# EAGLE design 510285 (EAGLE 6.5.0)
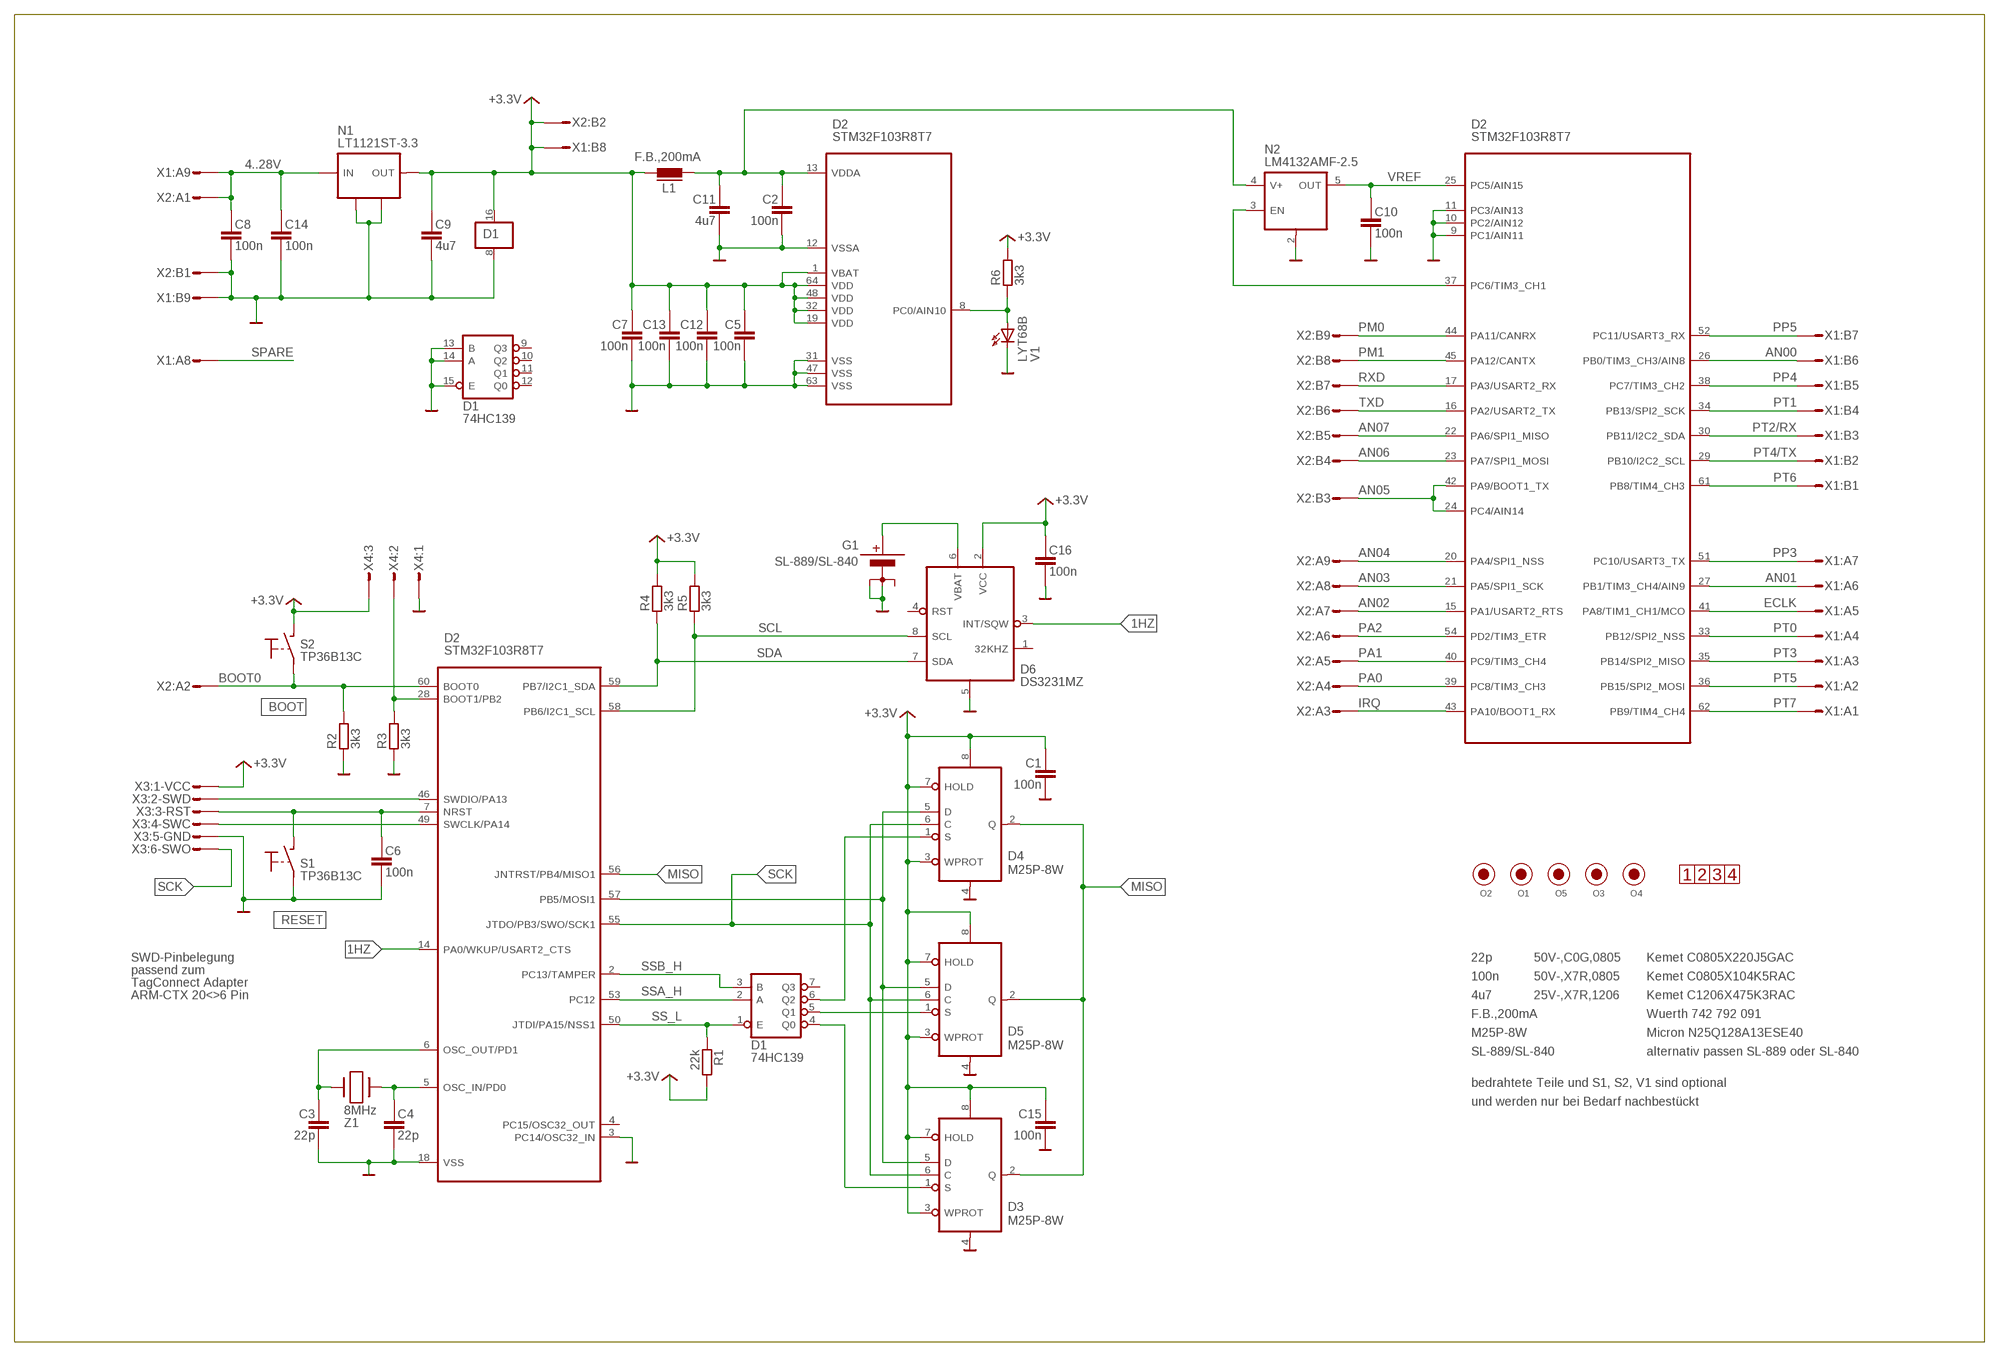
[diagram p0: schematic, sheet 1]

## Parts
C1  100n  C-EU-H-0805  [C0805]
C2  100n  C-EU-H-0805  [C0805]
C3  22p  C-EU-H-0805  [C0805]
C4  22p  C-EU-H-0805  [C0805]
C5  100n  C-EU-H-0805  [C0805]
C6  100n  C-EU-H-0805  [C0805]
C7  100n  C-EU-H-0805  [C0805]
C8  100n  C-EU-H-0805  [C0805]
C9  4u7  C-EU-H-1206  [C1206]
C10  100n  C-EU-H-0805  [C0805]
C11  4u7  C-EU-H-1206  [C1206]
C12  100n  C-EU-H-0805  [C0805]
C13  100n  C-EU-H-0805  [C0805]
C14  100n  C-EU-H-0805  [C0805]
C15  100n  C-EU-H-0805  [C0805]
C16  100n  C-EU-H-0805  [C0805]
D1  74HC139  74HC139D  [SO-16]
D2  STM32F103R8T7  [LQFP-10X10-64]
D3  M25P-8W  M25-8W  [SO-8-208MIL]
D4  M25P-8W  M25-8W  [SO-8-208MIL]
D5  M25P-8W  M25-8W  [SO-8-208MIL]
D6  DS3231MZ  [SO-8]
G1  SL-889/SL-840  BATTERIE-3MINUS  [SL-889/840-510285]
L1  F.B.,200mA  EMV-FERRIT-0805  [L0805]
N1  LT1121ST-3.3  [SOT-223]
N2  LM4132AMF-2.5  [MF05A]
O1  FIDUCIAL  [FIDUCIAL-1]
O2  FIDUCIAL  [FIDUCIAL-1]
O3  FIDUCIAL  [FIDUCIAL-1]
O4  FIDUCIAL  [FIDUCIAL-1]
O5  FIDUCIAL  [FIDUCIAL-1]
O6  1234-15  [1234-15]
R1  22k  R_0805  [R0805]
R2  3k3  R_0805  [R0805]
R3  3k3  R_0805  [R0805]
R4  3k3  R_0805  [R0805]
R5  3k3  R_0805  [R0805]
R6  3k3  R_0805  [R0805]
S1  TP36B13C  [TP36]
S2  TP36B13C  [TP36]
V1  LYT68B  LYT679-CO  [PLCC-2]
X1  1022-A-xx1-018  MODU-2X09-MVSS  [1022-A-XX1-018]
X2  1022-A-xx1-018  MODU-2X09-MVSS  [1022-A-XX1-018]
X3  SLR2-2x03  TAG-CONNECT-6M-SLR  [TAG-CONNECT-6-SLR]
X4  MODU-1X03-MV  [MODU-1X03-XV]
Z1  8MHz  HC-49/US-0.7  [HC-49/US-0.7]

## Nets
1HZ: D2.14(PA0/WKUP/USART2_CTS:I/O) D6.3(INT/SQW)
4..28V: C8.1 C14.1 N1.1(IN) X1.A9 X2.A1
+3.3V: C1.1 C5.1 C7.1 C9.1 C12.1 C13.1 C15.1 C16.1 D1.16(VDD) D2.1(VBAT:PWR) D2.19(VDD@19:VDD) D2.32(VDD@32:VDD) D2.48(VDD@48:VDD) D2.64(VDD@64:VDD) D3.3(WPROT) D3.7(HOLD) D3.8(VDD) D4.3(WPROT) D4.7(HOLD) D4.8(VDD) D5.3(WPROT) D5.7(HOLD) D5.8(VDD) D6.2(VCC) L1.1 N1.3(OUT) R1.2 R4.2 R5.2 R6.2 S2.1(NO1) X1.B8 X2.B2 X3.1 X4.3
AN00: D2.26(PB0/TIM3_CH3/AIN8:I/O) X1.B6
AN01: D2.27(PB1/TIM3_CH4/AIN9:I/O) X1.A6
AN02: D2.15(PA1/USART2_RTS:I/O) X2.A7
AN03: D2.21(PA5/SPI1_SCK:I/O) X2.A8
AN04: D2.20(PA4/SPI1_NSS:I/O) X2.A9
AN05: D2.24(PC4/AIN14:I/O) D2.42(PA9/BOOT1_TX:I/O) X2.B3
AN06: D2.23(PA7/SPI1_MOSI:I/O) X2.B4
AN07: D2.22(PA6/SPI1_MISO:I/O) X2.B5
BOOT0: D2.60(BOOT0:IN) R2.2 S2.2(NO2) X2.A2
BOOT1: D2.28(BOOT1/PB2:I/O) R3.2 X4.2
ECLK: D2.41(PA8/TIM1_CH1/MCO:I/O) X1.A5
GND: C1.2 C2.2 C3.2 C4.2 C5.2 C6.2 C7.2 C8.2 C9.2 C10.2 C11.2 C12.2 C13.2 C14.2 C15.2 C16.2 D1.8(GND) D1.13(B) D1.14(A) D1.15(E) D2.3(PC14/OSC32_IN:IN) D2.9(PC1/AIN11:I/O) D2.10(PC2/AIN12:I/O) D2.11(PC3/AIN13:I/O) D2.12(VSSA:PWR) D2.18(VSS@18:VSS) D2.31(VSS@31:VSS) D2.47(VSS@47:VSS) D2.63(VSS@63:VSS) D3.4(GND) D4.4(GND) D5.4(GND) D6.5(GND) G1.-2 G1.-BELP(-3) N1.2(GND) N1.4(GND) N2.2(GND) R2.1 R3.1 S1.2(NO2) V1.C X1.B9 X2.B1 X3.5 X4.1
IRQ: D2.43(PA10/BOOT1_RX:I/O) X2.A3
LED: D2.8(PC0/AIN10:I/O) R6.1 V1.A
MISO: D2.56(JNTRST/PB4/MISO1:I/O) D3.2(Q) D4.2(Q) D5.2(Q)
MOSI: D2.57(PB5/MOSI1:I/O) D3.5(D) D4.5(D) D5.5(D)
OSCIN: C4.1 D2.5(OSC_IN/PD0:IN) Z1.2
OSCOUT: C3.1 D2.6(OSC_OUT/PD1:OUT) Z1.1
PA0: D2.39(PC8/TIM3_CH3:I/O) X2.A4
PA1: D2.40(PC9/TIM3_CH4:I/O) X2.A5
PA2: D2.54(PD2/TIM3_ETR:I/O) X2.A6
PM0: D2.44(PA11/CANRX:I/O) X2.B9
PM1: D2.45(PA12/CANTX:I/O) X2.B8
PP3: D2.51(PC10/USART3_TX:I/O) X1.A7
PP4: D2.38(PC7/TIM3_CH2:I/O) X1.B5
PP5: D2.52(PC11/USART3_RX:I/O) X1.B7
PT0: D2.33(PB12/SPI2_NSS:I/O) X1.A4
PT1: D2.34(PB13/SPI2_SCK:I/O) X1.B4
PT2/RX: D2.30(PB11/I2C2_SDA:I/O) X1.B3
PT3: D2.35(PB14/SPI2_MISO:I/O) X1.A3
PT4/TX: D2.29(PB10/I2C2_SCL:I/O) X1.B2
PT5: D2.36(PB15/SPI2_MOSI:I/O) X1.A2
PT6: D2.61(PB8/TIM4_CH3:I/O) X1.B1
PT7: D2.62(PB9/TIM4_CH4:I/O) X1.A1
RESET_L: C6.1 D2.7(NRST:I/O) S1.1(NO1) X3.3
RXD: D2.17(PA3/USART2_RX:I/O) X2.B7
SCK: D2.55(JTDO/PB3/SWO/SCK1:I/O) D3.6(C) D4.6(C) D5.6(C) X3.6
SCL: D2.58(PB6/I2C1_SCL:I/O) D6.8(SCL) R5.1
SDA: D2.59(PB7/I2C1_SDA:I/O) D6.7(SDA) R4.1
SPARE: X1.A8
SS0_L: D1.4(Q0) D3.1(S)
SS1_L: D1.5(Q1) D5.1(S)
SS2_L: D1.6(Q2) D4.1(S)
SS_L: D1.1(E) D2.50(JTDI/PA15/NSS1:I/O) R1.1
SSA_H: D1.2(A) D2.53(PC12:I/O)
SSB_H: D1.3(B) D2.2(PC13/TAMPER:I/O)
SWCLK: D2.49(SWCLK/PA14:I/O) X3.4
SWDIO: D2.46(SWDIO/PA13:I/O) X3.2
TXD: D2.16(PA2/USART2_TX:I/O) X2.B6
VBAT [VBAT]: D6.6(VBAT) G1.+
VDDA: C2.1 C11.1 D2.13(VDDA:I/O) L1.2 N2.4(V+)
VREF: C10.1 D2.25(PC5/AIN15:I/O) N2.5(OUT)
VREFEN_H: D2.37(PC6/TIM3_CH1:I/O) N2.3(EN)
Unconnected: D1.7(Q3) D1.9(Q3) D1.10(Q2) D1.11(Q1) D1.12(Q0) D2.4(PC15/OSC32_OUT:OUT) D6.1(32KHZ) D6.4(RST) G1.-1 O1.F O2.F O3.F O4.F O5.F

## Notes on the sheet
- BOOT
- RESET
- SWD-Pinbelegung | 22p | 50V-,C0G,0805 | Kemet C0805X220J5GAC
- passend zum
- 100n | 50V-,X7R,0805 | Kemet C0805X104K5RAC
- TagConnect Adapter
- ARM-CTX 20<>6 Pin | 4u7 | 25V-,X7R,1206 | Kemet C1206X475K3RAC
- F.B.,200mA | Wuerth 742 792 091
- M25P-8W | Micron N25Q128A13ESE40
- SL-889/SL-840 | alternativ passen SL-889 oder SL-840
- bedrahtete Teile und S1, S2, V1 sind optional
- und werden nur bei Bedarf nachbestückt

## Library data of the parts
C1-C16 = din-C:C-EU-H-
D1 = din-D:74*139
D2 = din-D:STM32F103R
D3-D5 = din-D:M25*
D6 = din-D:DS3231*Z
G1 = din-G:BATTERIE-3MINUS
L1 = din-L:EMV-FERRIT: 0805: WE742792091, 1500Ohm@100MHz, 0.55Ohm, 0.2A
N1 = din-N:LT1121*
N2 = din-N:LM4132
O1-O5 = din-O:FIDUCIAL
O6 = din-O:1234
R1-R6 = din-R:R_
S1 S2 = din-S:TP36
V1 = din-V:L*T679-CO
X1 X2 = din-X:MODU-2X09-M
X3 = din-X:TAG-CONNECT-6M
X4 = din-X:MODU-1X03-M
Z1 = din-Z:HC-49/US

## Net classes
1 VBAT: clearance 0.53 mm to class 0

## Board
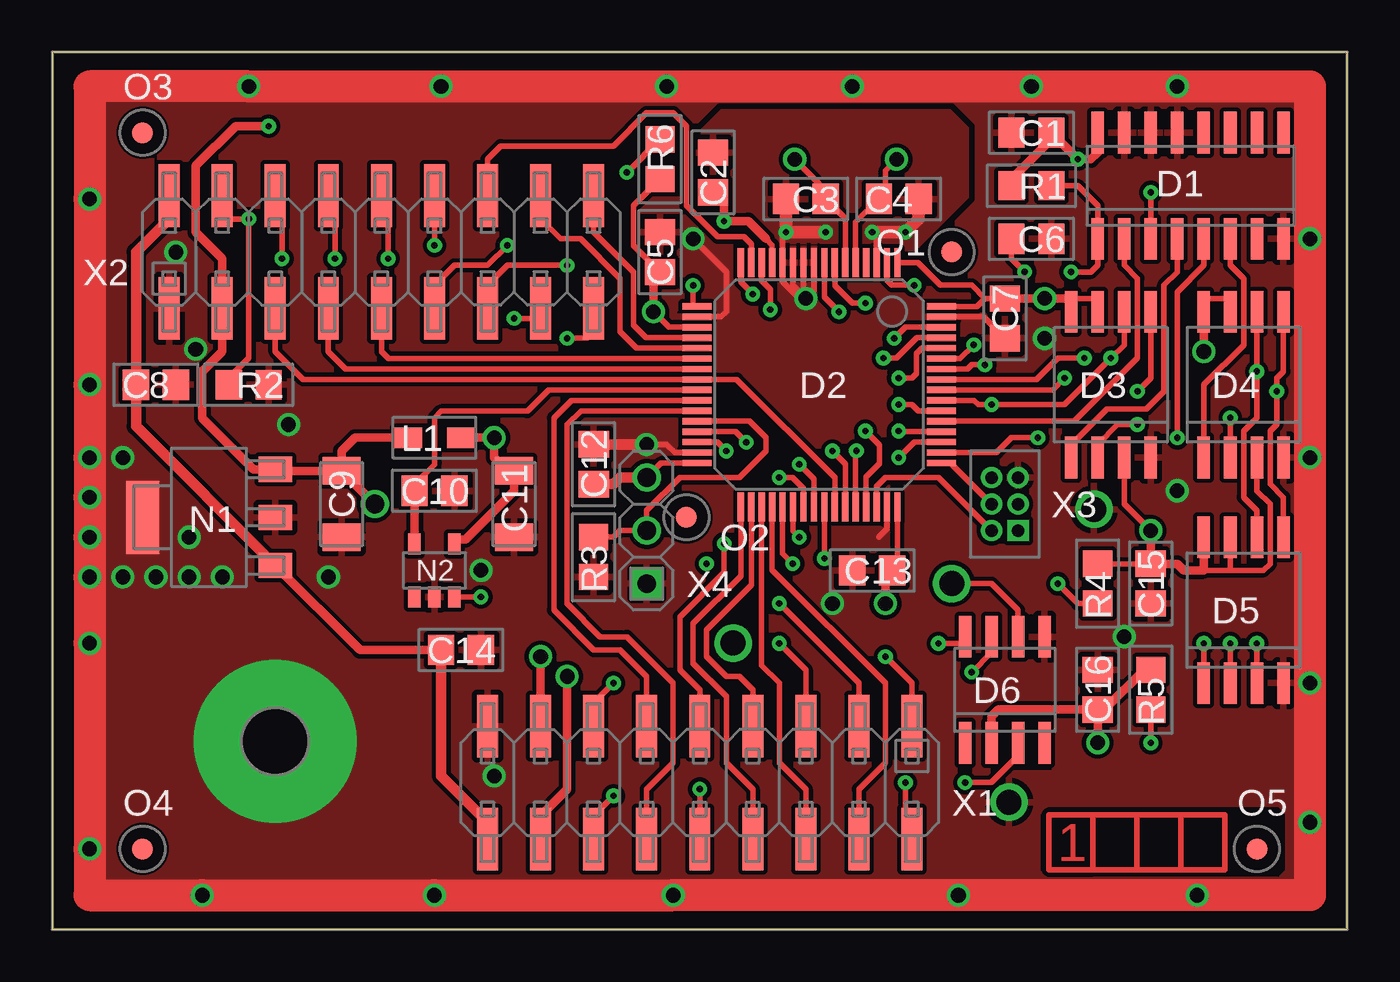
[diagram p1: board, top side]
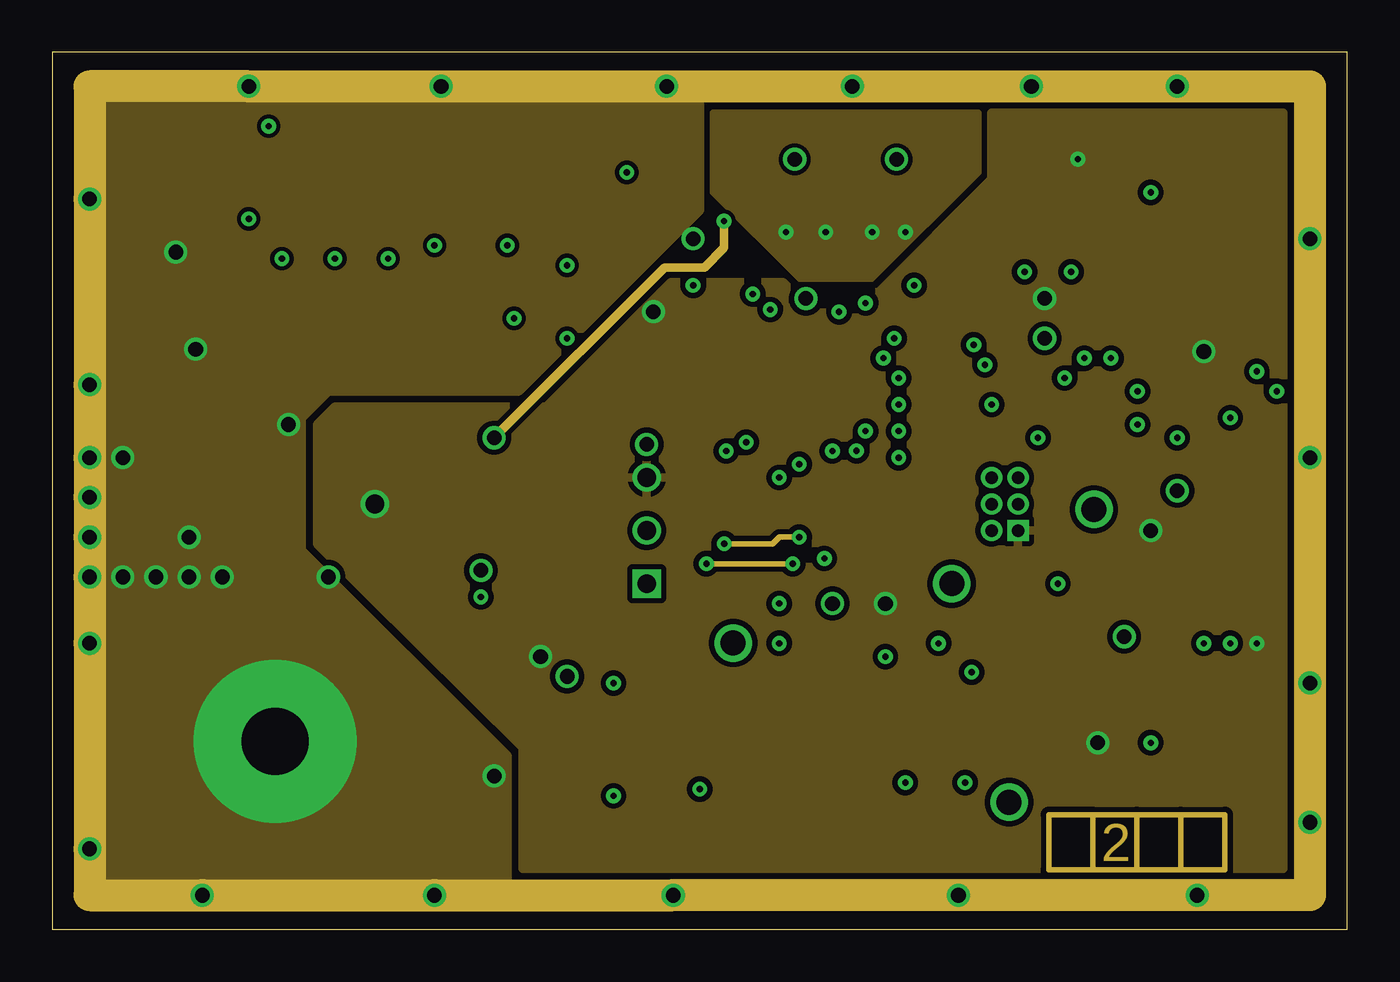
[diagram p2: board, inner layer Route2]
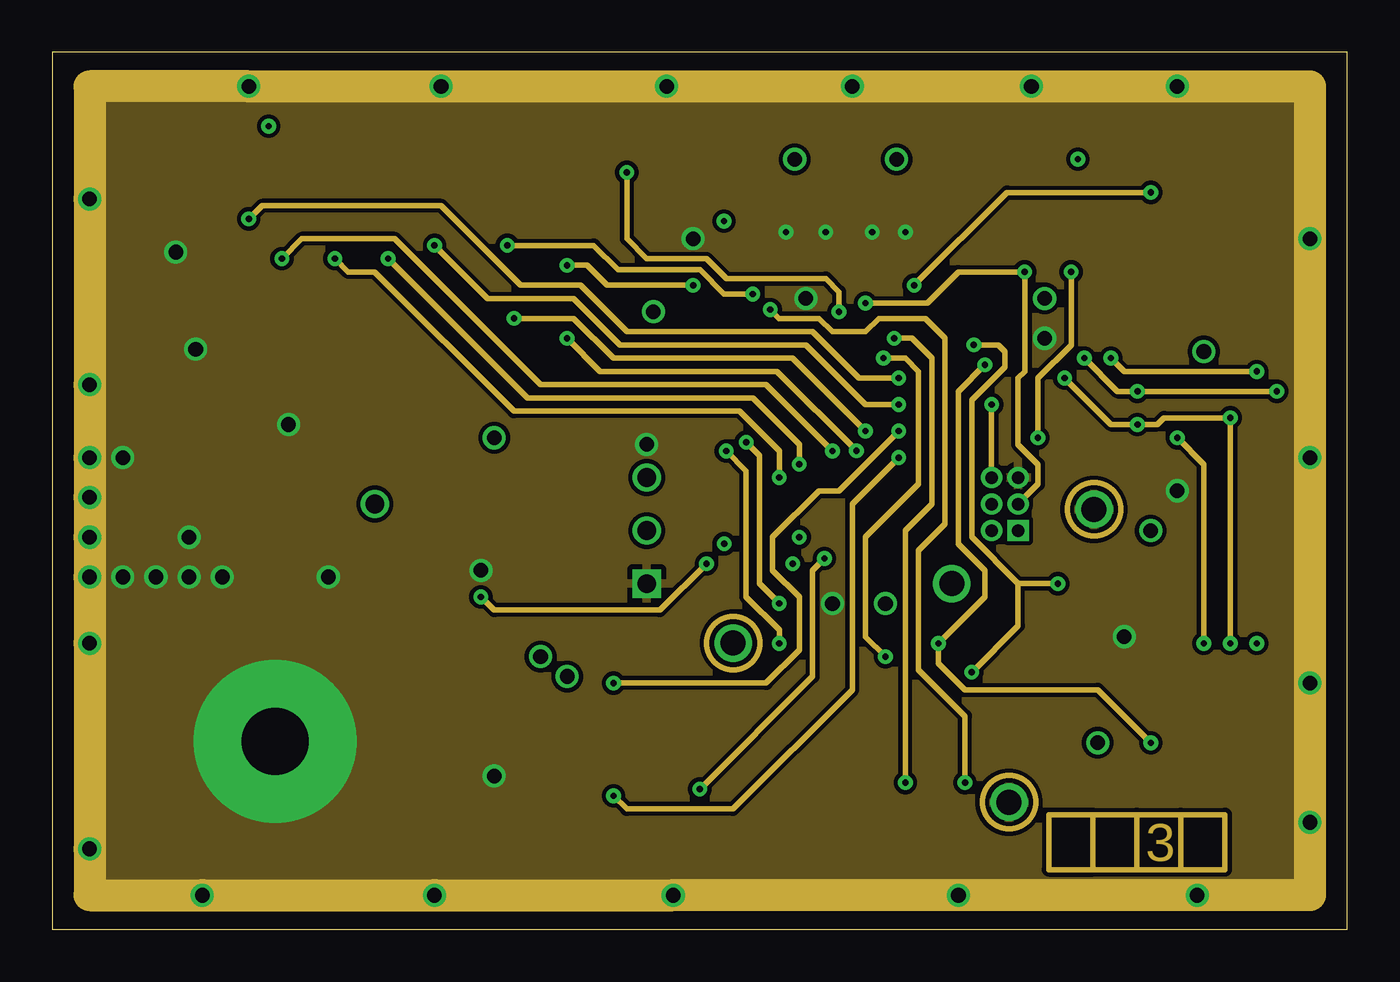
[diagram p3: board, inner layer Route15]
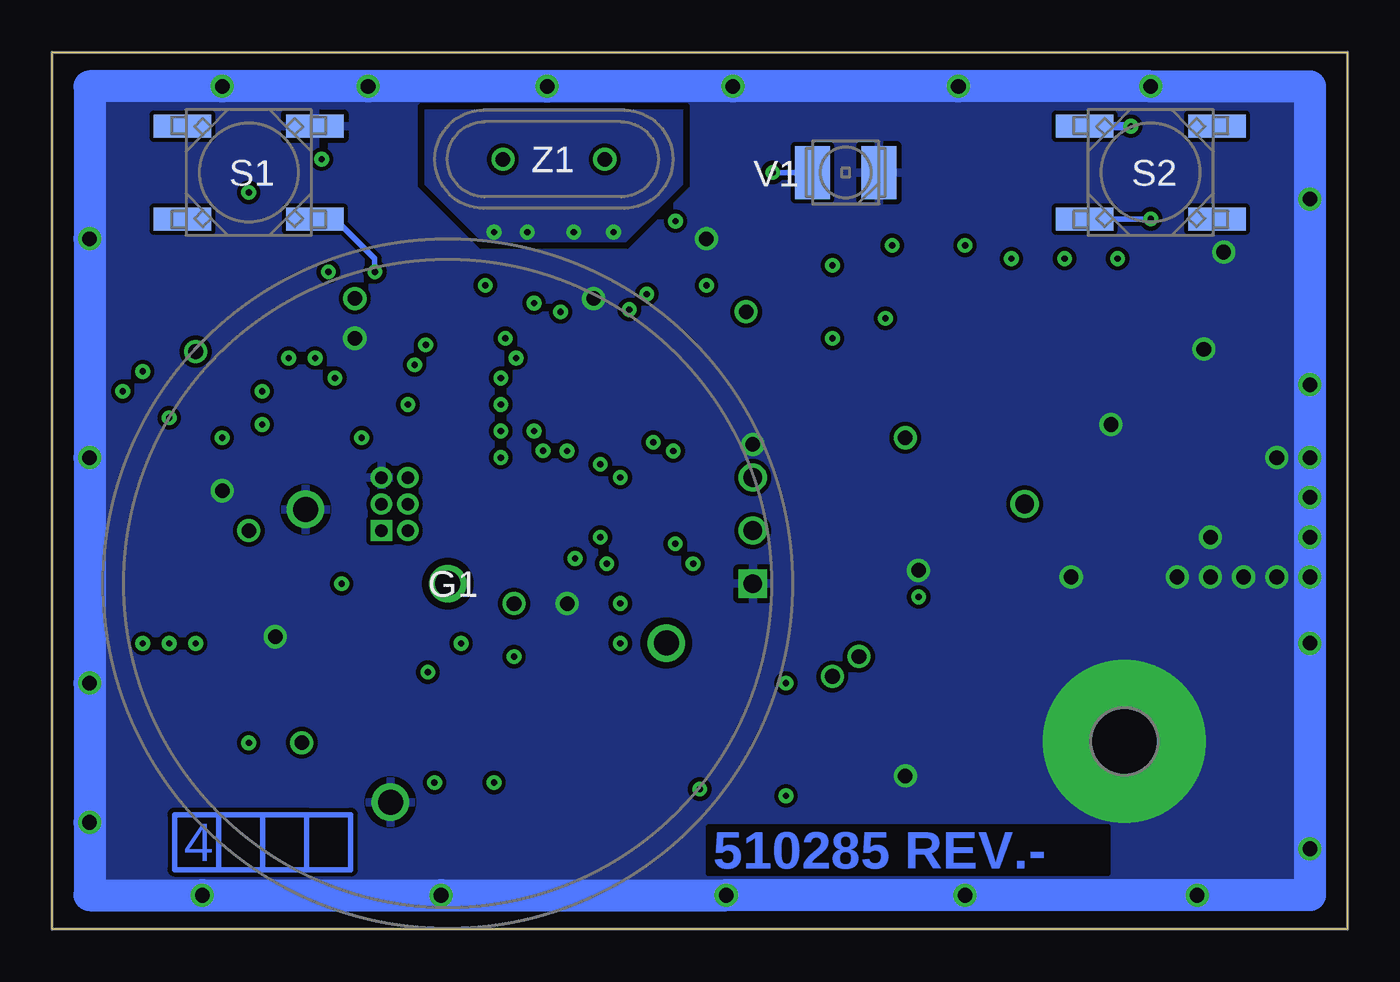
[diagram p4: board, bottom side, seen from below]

Size 62 x 42 mm. Coordinates in mm from the lower left corner, seen from the top.
Outline: 0,0 62,0 62,42 0,42 0,0
Copper layers (1+2*15+16): Top 0.018mm / dielectric 0.156mm / Route2 0.035mm / dielectric 1.2mm / Route15 0.035mm / dielectric 0.156mm / Bottom 0.018mm
Design rules "default *": minimum track width 10mil, minimum drill 0.3mm, track to track 8mil, track to pad 8mil, pad to pad 0.192mm, via to via 8mil, smd to smd 0.192mm, copper to edge 0.6mm, drill to drill 8mil, minimum pad ring 8mil, minimum via ring 8mil, stop-mask expansion 4mil, vias tented up to drill 0mil, thermal gap 10mil
tKeepout: area 2,4 to 14,10; area 5,3.2 to 16.4,14.6; area 50.1,3.9 to 60.2,8.9
tRestrict: 23 lines
bRestrict: 10 lines

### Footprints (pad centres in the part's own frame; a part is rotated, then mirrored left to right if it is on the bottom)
C0805 = smd 1.255 x 1.45: 1 -0.953,0; 2 0.953,0
C1206 = smd 1.325 x 1.8: 1 -1.587,0; 2 1.587,0
SO-16 = smd 0.6 x 2: 1 -4.445,-2.54; 2 -3.175,-2.54; 3 -1.905,-2.54; 4 -0.635,-2.54; 5 0.635,-2.54; 6 1.905,-2.54; 7 3.175,-2.54; 8 4.445,-2.54; 9 4.445,2.54; 10 3.175,2.54; 11 1.905,2.54; 12 0.635,2.54; 13 -0.635,2.54; 14 -1.905,2.54; 15 -3.175,2.54; 16 -4.445,2.54
LQFP-10X10-64 = smd 1.4 x 0.3: 1 -5.85,3.75; 2 -5.85,3.25; 3 -5.85,2.75; 4 -5.85,2.25; 5 -5.85,1.75; 6 -5.85,1.25; 7 -5.85,0.75; 8 -5.85,0.25; 9 -5.85,-0.25; 10 -5.85,-0.75; 11 -5.85,-1.25; 12 -5.85,-1.75; 13 -5.85,-2.25; 14 -5.85,-2.75; 15 -5.85,-3.25; 16 -5.85,-3.75; 33 5.85,-3.75; 34 5.85,-3.25; 35 5.85,-2.75; 36 5.85,-2.25; 37 5.85,-1.75; 38 5.85,-1.25; 39 5.85,-0.75; 40 5.85,-0.25; 41 5.85,0.25; 42 5.85,0.75; 43 5.85,1.25; 44 5.85,1.75; 45 5.85,2.25; 46 5.85,2.75; 47 5.85,3.25; 48 5.85,3.75 | smd 0.3 x 1.4: 17 -3.75,-5.85; 18 -3.25,-5.85; 19 -2.75,-5.85; 20 -2.25,-5.85; 21 -1.75,-5.85; 22 -1.25,-5.85; 23 -0.75,-5.85; 24 -0.25,-5.85; 25 0.25,-5.85; 26 0.75,-5.85; 27 1.25,-5.85; 28 1.75,-5.85; 29 2.25,-5.85; 30 2.75,-5.85; 31 3.25,-5.85; 32 3.75,-5.85; 49 3.75,5.85; 50 3.25,5.85; 51 2.75,5.85; 52 2.25,5.85; 53 1.75,5.85; 54 1.25,5.85; 55 0.75,5.85; 56 0.25,5.85; 57 -0.25,5.85; 58 -0.75,5.85; 59 -1.25,5.85; 60 -1.75,5.85; 61 -2.25,5.85; 62 -2.75,5.85; 63 -3.25,5.85; 64 -3.75,5.85
SO-8-208MIL = smd 0.6 x 2: 1 -1.905,-3.493; 2 -0.635,-3.493; 3 0.635,-3.493; 4 1.905,-3.493; 5 1.905,3.493; 6 0.635,3.493; 7 -0.635,3.493; 8 -1.905,3.493
SO-8 = smd 0.6 x 2: 1 -1.905,-2.54; 2 -0.635,-2.54; 3 0.635,-2.54; 4 1.905,-2.54; 5 1.905,2.54; 6 0.635,2.54; 7 -0.635,2.54; 8 -1.905,2.54
SL-889/840-510285 = drill 1.2: + 0,0; -1 10.465,-2.845; -2 -2.743,-10.465; -BELP -6.807,3.556
L0805 = smd 1.34 x 1: 1 -1.27,0; 2 1.27,0
SOT-223 = smd 1.2 x 1.6: 1 -2.3,-3.175; 2 0,-3.175; 3 2.3,-3.175 | smd 3.5 x 1.6: 4 0,3.175
MF05A = smd 0.6 x 1: 1 -0.953,-1.27; 2 0,-1.27; 3 0.953,-1.27; 4 0.953,1.27; 5 -0.953,1.27
FIDUCIAL-1 = smd 1 x 1: F 0,0
R0805 = smd 1.255 x 1.4: 1 -0.953,0; 2 0.953,0
TP36 = smd 1.1 x 2.75: 1 -2.223,-3.175; 2 2.223,-3.175; 3 2.223,3.175; 4 -2.223,3.175
PLCC-2 = smd 2.54 x 1.675: A 0,1.587; C 0,-1.587
1022-A-XX1-018 = smd 1 x 3: A1 -10.16,2.7; A2 -7.62,2.7; A3 -5.08,2.7; A4 -2.54,2.7; A5 0,2.7; A6 2.54,2.7; A7 5.08,2.7; A8 7.62,2.7; A9 10.16,2.7; B1 -10.16,-2.7; B2 -7.62,-2.7; B3 -5.08,-2.7; B4 -2.54,-2.7; B5 0,-2.7; B6 2.54,-2.7; B7 5.08,-2.7; B8 7.62,-2.7; B9 10.16,-2.7
TAG-CONNECT-6-SLR = drill 0.6 pad 1.016 square: 1 -1.27,-0.635 | drill 0.6 pad 1.016: 2 -1.27,0.635; 3 0,-0.635; 4 0,0.635; 5 1.27,-0.635; 6 1.27,0.635
MODU-1X03-XV = drill 0.9 square: 1 -2.54,0 | drill 0.9: 2 0,0; 3 2.54,0
HC-49/US-0.7 = drill 0.7 pad 1.1: 1 -2.44,0; 2 2.44,0

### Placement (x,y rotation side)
C1  46.88,38.14 180 top
C2  31.64,36.24 90 top
C3  36.08,34.97 180 top
C4  40.52,34.97 0 top
C5  29.09,32.43 90 top
C6  46.88,33.06 0 top
C7  45.61,29.26 270 top
C8  4.96,26.08 0 top
C9  13.86,20.36 270 top
C10  18.3,21 0 top
C11  22.11,20.36 270 top
C12  25.92,22.27 90 top
C13  39.26,17.19 180 top
C14  19.57,13.38 0 top
C15  52.59,16.55 270 top
C16  50.05,11.47 90 top
D1  54.5,35.61 0 top
D2  36.72,26.08 270 top
D3  50.69,26.08 0 top
D4  57.03,26.08 0 top
D5  57.03,15.29 0 top
D6  45.61,11.47 0 top
G1  43.06,16.55 0 bottom
L1  18.3,23.54 0 top
N1  7.5,19.73 90 top
N2  18.3,17.19 0 top
O1  43.06,32.43 0 top
O2  30.36,19.73 0 top
O3  4.33,38.14 0 top
O4  4.33,3.86 0 top
O5  57.67,3.86 0 top
O6  51.92,4.17 0 top
R1  46.88,35.61 180 top
R2  9.41,26.08 180 top
R3  25.92,17.82 90 top
R4  50.05,16.55 90 top
R5  52.59,11.47 90 top
R6  29.09,36.88 270 top
S1  52.59,36.24 90 bottom
S2  9.41,36.24 270 bottom
V1  24.02,36.24 90 bottom
X1  31,7.03 180 top
X2  15.76,32.43 0 top
X3  45.61,20.36 90 top
X4  28.46,19.09 90 top
Z1  37.98,36.88 180 bottom

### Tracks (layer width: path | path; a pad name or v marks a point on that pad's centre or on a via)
1HZ  (via drill 0.3)
  Top 0.254: D6.3 46.24,8.3 44.97,7.03 v43.7,7.03 | D2.14 33.97,31.05 34.38,30.64 v34.38,29.67
  Route15 0.254: v43.7,7.03 43.7,10.21 41.48,12.43 41.48,18.14 42.75,19.41 42.75,28.3 41.8,29.26 39.57,29.26 38.94,28.62 37.35,28.62 36.72,29.26 34.8,29.26 v34.38,29.67
4..28V
  Top 0.406: N1.1 14.73,13.38 C14.1
  Top 0.508: X2.A1 5.6,34.02 4.01,32.43 C8.1 4.01,24.1 N1.1 | X1.A9 20.84,5.12 18.62,7.35 C14.1
+3.3V  (via drill 0.3, 0.7, 0.9)
  Top 0.254: D2.48 40.47,17.45 C13.1 | D3.3 51.32,20.36 v52.59,19.09 | D2.64 44.27,29.83 44.65,30.21 | 44.65,30.21 C7.1 | D3.7 50.05,30.21 48.78,30.21 | D2.1 41.44,31.93 42.53,30.84 44.02,30.84 44.65,30.21 | D4.3 57.67,21 58.3,20.36 58.3,17.51 57.99,17.19 56.4,17.19 | 56.4,17.19 D5.7 | D4.7 56.4,30.21 55.13,30.21 D4.8 | 55.13,17.19 56.4,17.19 | D5.3 v57.67,13.7 | R4.2 C15.1 | D2.32 29.16,22.33 X4.3 | D2.19 29.52,28.83 v28.78,29.57 | R6.2 27.82,34.65 27.82,32.75 C5.1
  Top 0.406: v52.59,19.09 C15.1 53.86,17.51 54.18,17.19 55.13,17.19 D5.8 | v39.89,15.6 39.89,16.87 C13.1 | D6.2 44.97,10.21 45.29,10.52 C16.1 | C7.1 v47.51,30.21 48.78,30.21 D3.8 | R1.2 45.92,35.92 47.83,37.83 C1.1 v49.1,36.88 49.73,36.88 50.05,37.19 D1.16 | v55.13,27.67 D4.8 | C16.1 v50.05,8.94 | v28.78,29.57 28.78,31.16 C5.1 | C9.1 v15.44,20.36 | L1.1 14.49,23.54 13.86,22.91 C9.1 | v10.36,38.46 8.77,38.46 6.87,36.56 6.87,33.38 8.14,32.11 X2.B2 8.14,27.67 7.19,26.71 7.19,24.49 9.65,22.03 N1.3 10.76,21.95 C9.1 | R5.2 52.27,12.43 50.37,10.52 C16.1 | v23.38,13.06 X1.B8
  Top 0.508: X4.3 27.19,21.64 26.87,21.32 C12.1
  Bottom 0.406: S2.1 v10.36,38.46
  pour Route2 (isolate 0.254): 22.53,2.9 58.94,2.9 58.94,39.1 44.97,39.1 44.97,35.92 39.57,30.52 35.45,30.52 34.99,30.98 29.63,30.98 23.67,25.03 13.54,25.03 12.69,24.18 12.69,18.46 22.53,8.72
AN00
  Top 0.254: X1.B6 28.46,12.11 27.19,13.38 25.92,13.38 24.02,15.29 24.02,24.49 24.85,25.33 D2.26
AN01
  Top 0.254: X1.A6 28.46,6.71 29.73,7.98 29.73,11.79 27.51,14.02 26.24,14.02 24.65,15.6 24.65,24.18 25.3,24.83 D2.27
AN02
  Top 0.254: D2.15 33.47,32.82 33.12,33.17 31.85,33.17 30.36,34.65 30.36,38.46 29.73,39.1 28.46,39.1 26.87,37.51 21.48,37.51 20.84,36.88 X2.A7
AN03
  Top 0.254: D2.21 27.98,27.83 27.19,28.62 27.19,31.16 25.29,33.06 24.33,33.06 23.38,34.02 X2.A8
AN04
  Top 0.254: D2.20 28.43,28.33 27.82,28.94 27.82,31.48 25.92,33.38 X2.A9
AN05
  Top 0.254: X2.B3 10.68,27.67 12.02,26.33 D2.24 32.77,26.33 37.47,21.63 D2.42
AN06
  Top 0.254: D2.23 14.06,26.83 13.22,27.67 X2.B4
AN07
  Top 0.254: D2.22 16.1,27.33 15.76,27.67 X2.B5
BOOT0  (via drill 0.3)
  Top 0.254: D2.60 41.64,27.83 41.38,27.57 41.38,26.61 41.16,26.4 v40.52,26.4 | R2.2 8.46,26.4 9.41,27.35 v9.41,34.02 8.39,34.02 8.14,34.27 X2.A2
  Route15 0.254: v40.52,26.4 38.62,26.4 36.4,28.62 27.51,28.62 25.29,30.84 22.43,30.84 18.62,34.65 10.05,34.65 v9.41,34.02
  Bottom 0.254: v9.41,34.02 S2.2
BOOT1
  Top 0.254: R3.2 26.87,18.78 27.19,19.09 X4.2 28.46,20.05 30.05,21.64 32.91,21.64 34.17,22.91 34.17,23.54 33.38,24.33 D2.28
ECLK  (via drill 0.3)
  Top 0.254: v36.97,17.76 D2.41 | v31,6.71 X1.A5
  Route15 0.254: v36.97,17.76 36.4,17.19 36.4,12.11 v31,6.71
GND  (via drill 0.3, 0.7, 3.2 pad 7.8)
  Top 0.254: D2.47 39.97,19.17 39.57,18.78 | v36.08,30.21 35.76,30.21 34.97,31.01 D2.12 34.97,33.22 v35.13,33.38 | D2.9 36.47,30.59 v36.08,30.21 | D2.10 35.97,30.32 v36.08,30.21 | D2.11 35.47,30.82 v36.08,30.21 | D2.18 32.03,29.33 32.27,29.57 32.27,31.48 v30.68,33.06 | D2.3 39.47,33.17 v39.26,33.38 | D2.31 29.8,22.83 29.41,23.22 v28.46,23.22 | D2.63 44.58,29.33 C7.2
  Top 0.508: v28.46,23.22 C12.2
  Top 0.61: v39.26,33.38 v40.84,33.38 41.48,34.02 C4.2 41.48,35.29 | 35.13,35.29 C3.2 v35.13,33.38 v37.03,33.38
  Top 1.524: v1.79,13.7 v1.79,3.86 1.79,1.63 v7.19,1.63 v18.3,1.63 v29.73,1.63 v43.38,1.63 v54.81,1.63 60.21,1.63 v60.21,5.12 v60.21,11.79 v60.21,22.59 v60.21,33.06 60.21,40.37 v53.86,40.37 v46.88,40.37 v38.3,40.37 v29.41,40.37 v18.62,40.37 v9.41,40.37 1.79,40.37 v1.79,34.97 v1.79,26.08 v1.79,22.59 v1.79,20.68 v1.79,18.78 v1.79,16.87 v1.79,13.7
  Route2 1.524: v43.38,1.63 v29.73,1.63 v18.3,1.63 v7.19,1.63 1.79,1.63 v1.79,3.86 v1.79,13.7 v1.79,16.87 v1.79,18.78 v1.79,20.68 v1.79,22.59 v1.79,26.08 v1.79,34.97 1.79,40.37 v9.41,40.37 v18.62,40.37 v29.41,40.37 v38.3,40.37 v46.88,40.37 v53.86,40.37 60.21,40.37 v60.21,33.06 v60.21,22.59 v60.21,11.79 v60.21,5.12 60.21,1.63 v54.81,1.63 v43.38,1.63
  Route15 1.524: v1.79,34.97 v1.79,26.08 v1.79,22.59 v1.79,20.68 v1.79,18.78 v1.79,16.87 v1.79,13.7 v1.79,3.86 1.79,1.63 v7.19,1.63 v18.3,1.63 v29.73,1.63 v43.38,1.63 v54.81,1.63 60.21,1.63 v60.21,5.12 v60.21,11.79 v60.21,22.59 v60.21,33.06 60.21,40.37 v53.86,40.37 v46.88,40.37 v38.3,40.37 v29.41,40.37 v18.62,40.37 v9.41,40.37 1.79,40.37 v1.79,34.97
  Bottom 1.524: v1.79,26.08 v1.79,22.59 v1.79,20.68 v1.79,18.78 v1.79,16.87 v1.79,13.7 v1.79,3.86 1.79,1.63 v7.19,1.63 v18.3,1.63 v29.73,1.63 v43.38,1.63 v54.81,1.63 60.21,1.63 v60.21,5.12 v60.21,11.79 v60.21,22.59 v60.21,33.06 60.21,40.37 v53.86,40.37 v46.88,40.37 v38.3,40.37 v29.41,40.37 v18.62,40.37 v9.41,40.37 1.79,40.37 v1.79,34.97 v1.79,26.08
  other vias: 51.32,14.02 10.68,9 47.51,28.3 37.35,15.6 53.86,21 20.52,17.19 11.32,24.18 3.38,16.87 4.96,16.87 6.55,16.87 3.38,22.59 8.14,16.87 13.22,16.87 6.87,27.78 21.16,7.35 5.92,32.43 6.55,18.78
  pour Route2: 35.76,31.16 39.26,31.16 44.34,36.24 44.34,39.1 31.64,39.1 31.64,35.29
  pour Top: 1.79,1.63 60.21,1.63 60.21,40.37 1.79,40.37
  pour Bottom: 1.79,1.63 18.3,1.63 60.21,1.63 60.21,40.37 1.79,40.37
  pour Route15: 1.79,1.63 60.21,1.63 60.21,40.37 1.79,40.37
  pour Route2: 1.79,1.63 21.79,1.63 21.79,8.3 11.95,18.14 11.95,24.49 13.22,25.76 22.33,25.76 31,34.44 31,40.37 1.79,40.37
IRQ  (via drill 0.3)
  Top 0.254: D2.43 37.97,22.29 v37.35,22.91 | v11,32.11 11,34.34 10.68,34.65 X2.A3
  Route15 0.254: v37.35,22.91 34.17,26.08 23.38,26.08 16.39,33.06 11.95,33.06 v11,32.11
LED  (via drill 0.3)
  Top 0.254: D2.8 36.97,30.27 v37.67,29.57 | v27.51,36.24 R6.1
  Route15 0.254: v37.67,29.57 37.67,30.52 37.03,31.16 32.27,31.16 31.32,32.11 28.46,32.11 27.51,33.06 v27.51,36.24
  Bottom 0.254: v27.51,36.24 V1.A
MISO  (via drill 0.3)
  Top 0.254: v56.4,24.49 D4.2 | v51.95,24.18 51,24.18 50.05,23.22 D3.2 | v56.4,13.7 D5.2 | D2.56 47.89,25.83 v48.46,26.4
  Route15 0.254: v56.4,13.7 v56.4,24.49 53.23,24.49 52.91,24.18 v51.95,24.18 50.69,24.18 v48.46,26.4
MOSI  (via drill 0.3)
  Top 0.254: D5.5 58.94,20.68 58.3,21.32 58.3,23.86 58.62,24.18 v58.62,25.76 58.62,26.4 58.94,26.71 D4.5 | v51.95,25.76 52.59,26.4 D3.5 | D2.57 47.12,26.33 48.14,27.35 v49.41,27.35
  Route15 0.254: v58.62,25.76 v51.95,25.76 51,25.76 v49.41,27.35
OSCIN
  Top 0.254: Z1.2 39.89,36.34 39.89,35.29 C4.1 38.47,33.86 D2.5
OSCOUT
  Top 0.254: Z1.1 36.72,35.7 36.72,35.29 C3.1 37.97,34.04 D2.6
PA0  (via drill 0.3)
  Top 0.254: D2.39 35.97,21.11 35.45,21.64 v34.81,21.64 | v13.54,32.11 13.54,34.34 13.22,34.65 X2.A4
  Route15 0.254: v34.81,21.64 34.81,22.91 32.91,24.81 22.11,24.81 15.44,31.48 14.17,31.48 v13.54,32.11
PA1  (via drill 0.3)
  Top 0.254: D2.40 36.47,21.57 v35.76,22.27 | X2.A5 15.76,34.65 16.08,34.34 v16.08,32.11
  Route15 0.254: v35.76,22.27 35.76,23.22 33.54,25.45 22.74,25.45 v16.08,32.11
PA2  (via drill 0.3)
  Top 0.254: D2.54 41.46,24.83 41.16,25.13 v40.52,25.13 | X2.A6 v18.3,32.75
  Route15 0.254: v40.52,25.13 38.94,25.13 36.08,27.98 27.19,27.98 24.97,30.21 20.84,30.21 v18.3,32.75
PM0  (via drill 0.3)
  Top 0.254: X2.B9 25.92,28.62 25.6,28.3 v24.65,28.3 | D2.44 38.47,22.86 38.51,22.9 v38.51,22.92
  Route15 0.254: v24.65,28.3 26.24,26.71 34.71,26.71 v38.51,22.92
PM1  (via drill 0.3)
  Top 0.254: v38.94,23.86 39.6,23.2 39.6,22.3 38.97,21.66 D2.45 | X2.B8 23.38,29.26 v22.11,29.26
  Route15 0.254: v22.11,29.26 24.97,29.26 26.87,27.35 35.45,27.35 v38.94,23.86
PP3  (via drill 0.3)
  Top 0.254: D2.51 41.27,23.33 v40.52,22.59 | v26.87,6.39 25.92,5.44 X1.A7
  Route15 0.254: v40.52,22.59 38.3,20.36 38.3,11.47 32.59,5.76 27.51,5.76 v26.87,6.39
PP4  (via drill 0.3)
  Top 0.254: v32.17,18.46 32.17,17.09 30.05,14.97 30.05,12.43 31,11.47 X1.B5 | D2.38 35.47,19.07 v35.76,18.78
  Route2 0.254: v32.17,18.46 34.49,18.46 34.81,18.78 v35.76,18.78
PP5  (via drill 0.3)
  Top 0.254: D2.52 40.55,23.83 v40.52,23.86 | v26.87,11.79 25.92,10.84 X1.B7
  Route15 0.254: v40.52,23.86 37.67,21 36.72,21 34.49,18.78 34.49,17.19 35.76,15.92 35.76,13.38 34.17,11.79 v26.87,11.79
PT0
  Top 0.254: X1.A4 33.54,6.71 32.27,7.98 32.27,11.16 30.68,12.74 30.68,14.65 32.97,16.93 D2.33
PT1
  Top 0.254: X1.B4 33.54,11.47 32.91,12.11 32.27,12.11 31.32,13.06 31.32,14.33 33.47,16.48 D2.34
PT2/RX  (via drill 0.3)
  Top 0.254: v34.81,13.7 36.08,12.43 X1.B3 | D2.30 31.84,23.33 v32.27,22.91
  Route15 0.254: v34.81,13.7 34.81,14.33 33.22,15.92 33.22,21.95 v32.27,22.91
PT3
  Top 0.254: X1.A3 36.08,6.71 34.81,7.98 34.81,11.79 33.97,12.64 D2.35
PT4/TX  (via drill 0.3)
  Top 0.254: X1.B2 38.62,11.79 v34.81,15.6 | D2.29 32.72,23.83 v33.22,23.32
  Route15 0.254: v34.81,15.6 33.86,16.55 33.86,22.69 v33.22,23.32
PT5
  Top 0.254: X1.A2 38.62,6.71 39.89,7.98 39.89,11.79 34.47,17.22 D2.36
PT6  (via drill 0.3)
  Top 0.254: X1.B1 41.16,11.79 v39.89,13.06 | D2.61 41.39,28.33 40.41,27.35 v39.79,27.35
  Route15 0.254: v39.89,13.06 38.94,14.02 38.94,18.78 41.48,21.32 41.48,26.71 40.84,27.35 v39.79,27.35
PT7  (via drill 0.3)
  Top 0.254: D2.62 40.84,28.83 v40.31,28.3 | v40.84,7.03 40.84,4.65 X1.A1
  Route15 0.254: v40.84,7.03 40.84,19.09 42.11,20.36 42.11,27.35 41.16,28.3 v40.31,28.3
RESET_L  (via drill 0.3)
  Top 0.254: v46.56,31.48 45.92,32.11 C6.1 | D2.7 37.47,30.83 38.3,29.99 v38.94,29.99
  Route15 0.254: v38.94,29.99 41.9,29.99 43.38,31.48 v46.56,31.48 46.56,26.71 46.24,26.4 46.24,23.22 47.19,22.27 47.19,21.32 X3.3
  Bottom 0.254: v46.56,31.48 46.56,32.11 48.46,34.02 S1.1
RXD  (via drill 0.3)
  Top 0.254: X2.B7 20.84,30.84 21.79,31.8 v24.65,31.8 | D2.17 30.68,29.83 v30.68,30.84
  Route15 0.254: v30.68,30.84 26.55,30.84 25.6,31.8 v24.65,31.8
SCK  (via drill 0.3)
  Top 0.254: D2.55 44.13,25.33 44.34,25.13 v44.97,25.13 48.46,25.13 v50.69,27.35 51.32,27.98 D3.6 | D5.6 57.67,20.05 57.03,20.68 57.03,23.86 57.67,24.49 v57.67,26.71 D4.6
  Route15 0.254: v44.97,25.13 X3.6 | v50.69,27.35 51.32,26.71 v57.67,26.71
SCL  (via drill 0.3)
  Top 0.254: D2.58 43.81,26.83 44.02,27.03 v44.65,27.03 | D6.8 43.7,13.7 v42.43,13.7 | v52.59,8.94 R5.1
  Route15 0.254: v44.65,27.03 43.38,25.76 43.38,18.46 44.65,17.19 44.65,15.92 v42.43,13.7 42.43,12.74 43.7,11.47 50.05,11.47 v52.59,8.94
SDA  (via drill 0.3)
  Top 0.254: D2.59 43.46,27.33 v44.12,27.98 | v48.14,16.55 49.1,15.6 R4.1 | v44.02,12.31 44.97,13.27 D6.7
  Route15 0.254: v44.12,27.98 45.29,27.98 45.61,27.67 45.61,26.93 44.02,25.34 44.02,18.78 46.24,16.55 | 46.24,16.55 v48.14,16.55 | 46.24,16.55 46.24,14.54 v44.02,12.31
SPARE  (via drill 0.7)
  Top 0.406: X1.A8 23.38,5.44 24.65,6.71 v24.65,12.11
SS0_L
  Top 0.254: D1.4 53.86,31.48 53.23,30.84 53.23,25.76 52.39,24.92 50.48,24.92 48.78,23.22 D3.1
SS1_L  (via drill 0.3)
  Top 0.254: v53.86,23.54 53.86,30.52 55.13,31.8 D1.5 | D5.1 v55.13,13.7
  Route15 0.254: v55.13,13.7 55.13,22.27 v53.86,23.54
SS2_L
  Top 0.254: D4.1 55.13,26.08 57.03,27.98 57.03,31.16 56.4,31.8 D1.6
SS_L  (via drill 0.3)
  Top 0.254: D2.50 45.21,22.83 45.92,23.54 v47.19,23.54 | R1.1 49.1,35.61 50.05,34.65 D1.1 50.05,31.8 49.73,31.48 v48.78,31.48
  Route15 0.254: v48.78,31.48 48.78,27.98 47.19,26.4 v47.19,23.54
SSA_H
  Top 0.254: D1.2 51.32,31.8 51.95,31.16 51.95,27.35 48.94,24.33 D2.53
SSB_H  (via drill 0.3)
  Top 0.254: v52.59,35.29 D1.3 | D2.2 39.97,31.09 40.21,30.84 v41.26,30.84
  Route15 0.254: v52.59,35.29 45.71,35.29 v41.26,30.84
SWCLK
  Top 0.254: D2.49 43.01,22.33 X3.4
SWDIO
  Top 0.254: X3.2 42.43,21.64 39.89,21.64 39.47,21.21 D2.46
TXD  (via drill 0.3)
  Top 0.254: D2.16 32.97,31 v33.54,30.42 | v21.79,32.75 20.84,31.8 19.25,31.8 18.3,30.84 X2.B6
  Route15 0.254: v33.54,30.42 32.16,30.42 31,31.58 27.09,31.58 25.92,32.75 v21.79,32.75
VBAT
  Top 0.254: D6.6 46.24,15.29 44.97,16.55 G1.+
VDDA  (via drill 0.3, 0.7)
  Top 0.254: D2.13 34.47,32.77 34.17,33.06
  Top 0.406: 34.17,33.06 33.32,33.92 v32.16,33.92 32.16,34.77 C2.1 | N2.4 19.47,18.68 19.79,18.68 22.11,21 C11.1 21.79,21.95 21.16,22.59 v21.16,23.54 L1.2
  Route2 0.406: v32.16,33.92 32.16,32.63 31.22,31.69 29.31,31.69 v21.16,23.54
VREF
  Top 0.254: D2.25 23.77,25.83 22.74,24.81 18.62,24.81 18.3,24.49 18.3,22.27 17.35,21.32 C10.1
  Top 0.406: C10.1 N2.5
VREFEN_H  (via drill 0.3)
  Top 0.254: D2.37 34.97,17.99 v35.45,17.51 | v20.52,15.92 N2.3
  Route2 0.254: v35.45,17.51 v31.32,17.51
  Route15 0.254: v31.32,17.51 29.09,15.29 21.16,15.29 v20.52,15.92
(copper drawn outside any net)
  shapes: Route15 circle x3

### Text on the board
Bottom: 510285 REV.-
